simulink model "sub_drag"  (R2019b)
settings: Solver=VariableStepAuto  StartTime=0.0  StopTime=20  RelTol=1e-3
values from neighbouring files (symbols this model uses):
  A = 2.397    [EV_data.m]
  Cd = 0.308    [EV_data.m]
  mu_roll = 0.01    [EV_data.m]
undefined symbols (not defined in the file or in its folder): M_body
libraries: simulink x1

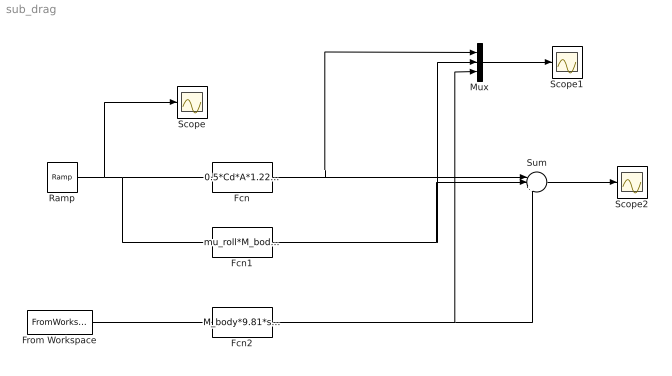
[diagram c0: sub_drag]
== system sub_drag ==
  Fcn : Fcn  Expr=0.5*Cd*A*1.226*u^2
  Fcn1 : Fcn  Expr=mu_roll*M_body*9.81*tanh(u)
  Fcn2 : Fcn  Expr=M_body*9.81*sin(u)
  From Workspace : FromWorkspace  VariableName=grad
  Mux : Mux  Inputs=3
  Ramp : simulink/Sources/Ramp  slope=2  start=1  InitialOutput=0
  Scope : Scope
  Scope1 : Scope
  Scope2 : Scope
  Sum : Sum  Inputs=|+++
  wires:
  Ramp/1 -> Scope/1, Fcn1/1, Fcn/1
  From Workspace/1 -> Fcn2/1
  Fcn/1 -> Sum/1, Mux/1
  Fcn1/1 -> Sum/2, Mux/2
  Fcn2/1 -> Mux/3, Sum/3
  Mux/1 -> Scope1/1
  Sum/1 -> Scope2/1
